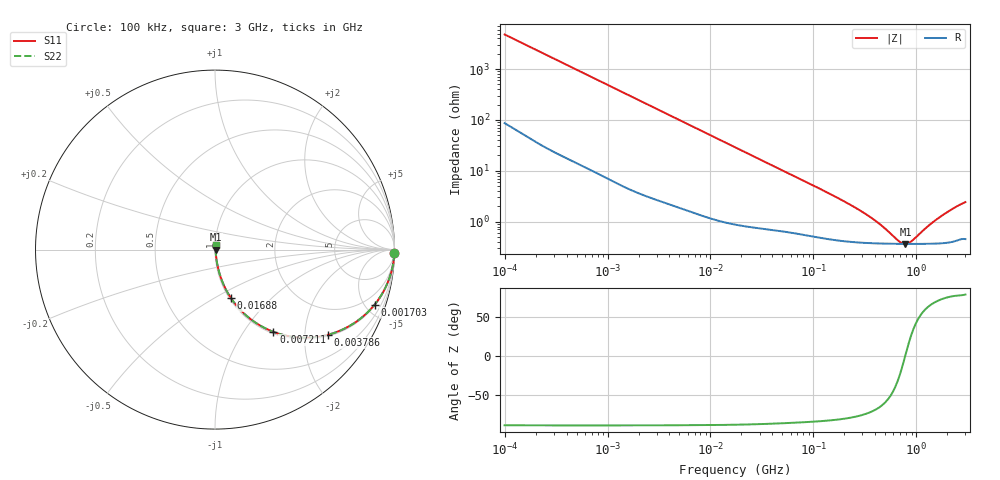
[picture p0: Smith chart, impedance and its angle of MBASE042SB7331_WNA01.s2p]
! MBASE042SB7331_WNA01  S-PARAMETER MODEL  ( Standard Model )
! Model Generated by TAIYO YUDEN Corporation (https://www.yuden.co.jp/en/)
! Version 1.0
! TAIYO YUDEN Control No. 250312
! Copyright(c) 2025 TAIYO YUDEN CO.,LTD. All Rights Reserved.
! Product Description (link to TY-COMPAS)
! https://ds.yuden.co.jp/TYCOMPAS/or/detail?pn=MBASE042SB7331KWNA01&u=M
! Products Name : Multilayer Ceramic Capacitors
! Characteristics :
!  Capacitance : 330 [pF] , Rated Voltage : 16 [V] , TCC : X7R
!  Case Size : 0.4 x 0.2 / 0.016 x 0.008 [mm/inch] , Thickness : 0.2 / 0.008 [mm/inch]
!  (Conditions: Temperature = 25 [degC] , DC Bias Voltage = 0 [V])
! External Node Assignments :
!  1  o---| |---o  2
! GND o---------o GND
! Frequency Range : 100kHz  -  3GHz  [ 401 STEP ]
# MHZ S RI R 50
! Freq[MHz].  S11 Real  S11 Imag  S21 Real  S21 Imag  S12 Real  S12 Imag  S22 Real  S22 Imag
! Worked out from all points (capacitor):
!   401 points, 100 kHz to 3 GHz, reference 50 ohm
!   read as one part in series: C = 331 pF near 105.3 kHz
!   lowest |Z| = 364 mohm at 785.4 MHz (marker M1)
!   series resonance near 779.7 MHz, so ESL is about 130 pH
!   S11 on the Smith chart (normalised r, x): 100 kHz: 3, -96; 1.703 MHz: 1.08, -5.77; 3.786 MHz: 1.05, -2.61; 7.211 MHz: 1.03, -1.38; 16.88 MHz: 1.02, -0.59; 3 GHz: 1.01, +0.05
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0.1  0.9992 -0.0208  0.000811 0.0208  0.000811 0.0208  0.9992 -0.0208
0.562235  0.9852 -0.1136  0.0148 0.1136  0.0148 0.1136  0.9852 -0.1136
1.070873  0.9517 -0.2075  0.0483 0.2075  0.0483 0.2075  0.9517 -0.2075
1.702975  0.8893 -0.3067  0.1107 0.3067  0.1107 0.3067  0.8893 -0.3067
3.161081  0.706 -0.4474  0.294 0.4474  0.294 0.4474  0.706 -0.4474
3.78604  0.6282 -0.4747  0.3718 0.4747  0.3718 0.4747  0.6282 -0.4747
5.158208  0.4806 -0.4902  0.5194 0.4902  0.5194 0.4902  0.4806 -0.4902
7.211163  0.3259 -0.4584  0.6741 0.4584  0.6741 0.4584  0.3259 -0.4584
10.89156  0.1794 -0.372  0.8206 0.372  0.8206 0.372  0.1794 -0.372
16.87982  0.0876 -0.2682  0.9124 0.2682  0.9124 0.2682  0.0876 -0.2682
17.7727  0.0803 -0.2569  0.9197 0.2569  0.9197 0.2569  0.0803 -0.2569
38.50681  0.0234 -0.1271  0.9766 0.1271  0.9766 0.1271  0.0234 -0.1271
97.38194  0.00777 -0.0517  0.9922 0.0517  0.9922 0.0517  0.00777 -0.0517
287.4592  0.00409 -0.0157  0.9959 0.0157  0.9959 0.0157  0.00409 -0.0157
412.3589  0.00379 -0.00916  0.9962 0.00916  0.9962 0.00916  0.00379 -0.00916
547.5153  0.00368 -0.00486  0.9963 0.00486  0.9963 0.00486  0.00368 -0.00486
690.4488  0.00363 -0.00164  0.9964 0.00164  0.9964 0.00164  0.00363 -0.00164
785.4083  0.00363 9.96e-05  0.9964 -9.96e-05  0.9964 -9.96e-05  0.00363 9.96e-05
893.4279  0.00363 0.00184  0.9964 -0.00184  0.9964 -0.00184  0.00363 0.00184
1315.078  0.0037 0.00739  0.9963 -0.00739  0.9963 -0.00739  0.0037 0.00739
1746.113  0.00387 0.0121  0.9961 -0.0121  0.9961 -0.0121  0.00387 0.0121
3000  0.00505 0.0235  0.9949 -0.0235  0.9949 -0.0235  0.00505 0.0235
